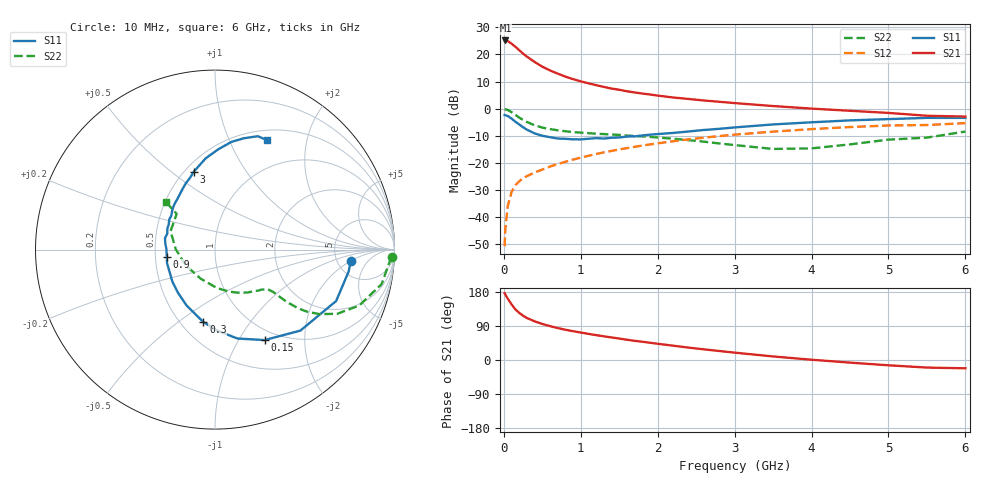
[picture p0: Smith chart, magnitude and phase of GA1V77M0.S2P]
! Infineon Technologies  Discrete & RF Semiconductors
! BF775
! Si NPN RF Bipolar Junction Transistor in SOT23
! VCE = 1.75 V  IC = 7 mA
! Common Emitter S-Parameters:  May  1996
# GHz  S  MA  R  50
!  f  S11  S21  S12  S22
! GHz  MAG  ANG  MAG  ANG  MAG  ANG  MAG  ANG
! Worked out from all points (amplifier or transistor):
!   36 points, 10 MHz to 6 GHz, reference 50 ohm
!   highest |S21| = 25.2 dB at 20 MHz (marker M1)
!   |S21| within 3 dB of that: start of sweep to 176.8 MHz
!   unconditionally stable (mu >= 1): 639.4 MHz to 4.053 GHz; 5.319 GHz to 5.818 GHz
!   at 250 MHz: K = 0.60, MSG = 23.0 dB, |S12| = -25.7 dB
!   at 1.4 GHz: K = 1.14, MAG = 9.2 dB, |S12| = -15.6 dB
!   at 6 GHz: K = 0.99, MSG = 1.2 dB, |S12| = -5.3 dB
!   S11 on the Smith chart (normalised r, x): 10 MHz: 6.70, -2.02; 150 MHz: 0.86, -1.30; 300 MHz: 0.64, -0.62; 900 MHz: 0.58, -0.05; 3 GHz: 0.55, +0.60; 6 GHz: 0.62, +1.40
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0.01  0.7597 -4.8  18.09 176.5  0.0029 84.1  0.9853 -2.4
0.02  0.7542 -9.4  18.12 172.5  0.0062 86.6  0.972 -4.7
0.05  0.7332 -23.0  17.66 162.2  0.0157 78.2  0.9479 -11.7
0.1  0.6557 -43.5  15.81 147.0  0.0289 68.9  0.8619 -21.2
0.15  0.5747 -61.3  13.87 133.6  0.0387 63.5  0.7694 -27.7
0.2  0.511 -75.8  12 124.4  0.0456 59.8  0.684 -31.7
0.25  0.4537 -88.0  10.36 116.9  0.0521 57.5  0.6187 -34.0
0.3  0.4089 -99.1  9.105 110.8  0.0569 57.4  0.5675 -35.2
0.4  0.3494 -117.0  7.269 102.1  0.0664 57.0  0.4938 -36.1
0.5  0.3162 -130.9  5.954 95.0  0.0752 57.7  0.4471 -36.1
0.6  0.2971 -143.1  5.077 89.4  0.0853 58.0  0.4196 -36.0
0.7  0.2809 -155.1  4.426 84.3  0.095 58.7  0.3987 -36.1
0.9  0.2714 -171.8  3.506 76.0  0.1149 59.2  0.3695 -36.9
1.1  0.2787 173.1  2.931 69.0  0.135 59.0  0.3528 -39.0
1.3  0.2805 161.6  2.516 62.5  0.1561 58.1  0.3393 -41.4
1.6  0.3055 146.3  2.093 53.5  0.187 56.1  0.3191 -46.3
2.2  0.3558 125.1  1.607 37.8  0.2502 50.7  0.2789 -59.6
3  0.4502 105.2  1.267 19.4  0.3316 41.1  0.2127 -87.9
3.5  0.5114 95.8  1.117 9.4  0.3768 34.5  0.1804 -116.4
4.5  0.6072 81.3  0.913 -6.9  0.4578 21.0  0.219 179.4
5.5  0.6753 69.3  0.739 -20.0  0.4988 6.7  0.292 137.0
6  0.6755 64.4  0.714 -21.9  0.5403 2.7  0.3778 135.9
